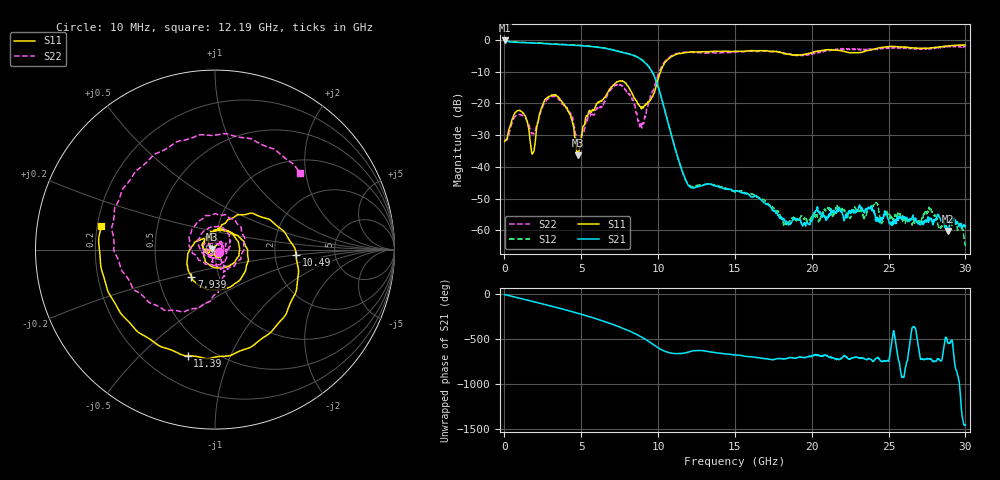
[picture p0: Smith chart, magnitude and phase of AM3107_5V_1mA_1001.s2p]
# Hz S DB R 50.0
!freq dBS11 angS11 dBS21 angS21 dBS12 angS12 dBS22 angS22
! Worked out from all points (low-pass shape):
!   1601 points, 10 MHz to 30 GHz, reference 50 ohm
!   highest |S21| = -0.15 dB at 10 MHz (marker M1); lowest = -60.2 dB at 28.86 GHz (marker M2)
!   |S21| within 3 dB of the highest: start of sweep to 7.033 GHz
!   lowest |S11| = -36.3 dB at 4.808 GHz (marker M3), VSWR 1.03, Z = 48.5 + j0.301 ohm
!   |S11| at or under -10 dB: start of sweep to 10.16 GHz
!   |S22| runs from -33.1 to -1.8 dB; largest |S21 - S12| = 0.016
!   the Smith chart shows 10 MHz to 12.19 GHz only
!   S11 on the Smith chart (normalised r, x): 10 MHz: 1.03, -0.04; 7.939 GHz: 0.74, -0.23; 10.49 GHz: 2.63, -0.20; 11.39 GHz: 0.37, -0.70; 12.19 GHz: 0.22, +0.10
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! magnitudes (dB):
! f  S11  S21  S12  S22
! 10 MHz  -31.9  -0.2  -0.2  -31.2
! 1.003 GHz  -22.2  -0.8  -0.7  -23.4
! 1.866 GHz  -35.5  -0.9  -0.8  -29.3
! 2.484 GHz  -20.4  -1.1  -1.0  -21.1
! 3.234 GHz  -17.3  -1.3  -1.3  -17.7
! 4.19 GHz  -22.7  -1.5  -1.5  -22.1
! 4.808 GHz  -36.3  -1.7  -1.6  -32.6
! 5.015 GHz  -29.9  -1.8  -1.7  -32.1
! 6.983 GHz  -14.8  -3.1  -3.0  -15.2
! 7.939 GHz  -13.9  -4.2  -4.1  -16.2
! 8.932 GHz  -21.5  -6.3  -6.2  -27.7
! 10.02 GHz  -12.1  -15.0  -14.8  -10.7
! 10.49 GHz  -6.9  -23.1  -23.0  -6.5
! 11.39 GHz  -4.3  -38.6  -38.7  -4.1
! 12.19 GHz  -3.8  -46.5  -46.1  -3.9
! 15.01 GHz  -3.6  -47.5  -47.9  -3.7
! 18.3 GHz  -4.4  -57.8  -57.8  -4.2
! 20.01 GHz  -4.0  -56.9  -55.7  -4.5
! 25.01 GHz  -2.1  -57.0  -54.8  -2.6
! 27.69 GHz  -2.5  -56.6  -53.9  -2.6
! 28.86 GHz  -1.9  -60.2  -59.7  -2.2
! 30 GHz  -1.5  -58.5  -64.9  -1.9
